(* Logix 5000 AddOnInstructionDefinition export V430_Trigger_Input_MXLSLC_102; software revision 33.01 *)

TYPE INPUT_MXLSLC_102 :
STRUCT
   Info : V430_InfoBits;
   Device_Status : V430_Device_Status;
   Fault_Code : DINT;
   Counters : V430_CodeReader_Counters;
   Read_Cycle_Report : V430_Read_Cycle_Report;
   Decode_Report : V430_Decode_Cycle_Report;
   Decode_Data : V430_MXLSLC_Str;
END_STRUCT
END_TYPE

TYPE OUTPUT_197 :
STRUCT
   Commands : V430_197_Commands;
END_STRUCT
END_TYPE

TYPE V430_197_Commands :
STRUCT
   Run_Mode : BOOL;
   Trigger : BOOL;
   Enable_Matchcode : BOOL;
   Reset_General_Fault : BOOL;
   Clear_NoRead_ReadCycle_Count : BOOL;
   Clear_MisMatch_ReadCycle_Count : BOOL;
   Clear_NoRead_Count : BOOL;
   Clear_Trigger_Count : BOOL;
   Clear_Matchcode_Count : BOOL;
   Clear_Mismatch_Count : BOOL;
   Output_1 : BOOL;
   Output_2 : BOOL;
   Output_3 : BOOL;
   Reserved1 : BOOL;
   Reserved2 : BOOL;
   Reserved3 : BOOL;
   Reserved4 : BOOL;
   Reserved5 : BOOL;
   Reserved6 : BOOL;
   Reserved7 : BOOL;
   Reserved8 : BOOL;
   Reserved9 : BOOL;
   Reserved10 : BOOL;
   Reserved11 : BOOL;
   Reserved12 : BOOL;
   Reserved13 : BOOL;
   Reserved14 : BOOL;
   Reserved15 : BOOL;
   Reserved16 : BOOL;
   Reserved17 : BOOL;
   Reserved18 : BOOL;
   Reserved19 : BOOL;
END_STRUCT
END_TYPE

TYPE V430_CodeReader_Counters :
STRUCT
   Noread_Read_Cycle_Counter : DINT;
   Mismatch_Per_Read_Cycle_Counter : DINT;
   No_Read_Counter : DINT;
   Trigger_Counter : DINT;
   Match_Code_Counter : DINT;
   Mismatch_Counter : DINT;
END_STRUCT
END_TYPE

TYPE V430_Decode_Cycle_Report :
STRUCT
   Decode_Location_Top : INT;
   Decode_Location_Left : INT;
   Decode_Location_Height : INT;
   Decode_Location_Width : INT;
   Code_Type : V430_Decode_Type;
   Pixels_Per_Element : REAL;
END_STRUCT
END_TYPE

TYPE V430_Decode_Type :
STRUCT
   Aztec : BOOL;
   MicroQR : BOOL;
   Postal_Code : BOOL;
   Code39 : BOOL;
   Codeabar : BOOL;
   I_2of5 : BOOL;
   UPC_EAN : BOOL;
   Code128_EAN128 : BOOL;
   Code93 : BOOL;
   PDF417 : BOOL;
   Pharmacode : BOOL;
   Data_Matrix : BOOL;
   QR_Code : BOOL;
   BC412 : BOOL;
   GS1_Databar : BOOL;
   GS1_Databar_Limited : BOOL;
   GS1_Databar_Expanded : BOOL;
   MicroPDF : BOOL;
   Composite : BOOL;
   Dot_Code : BOOL;
   Reserved_01 : BOOL;
   Reserved_02 : BOOL;
   Reserved_03 : BOOL;
   Reserved_04 : BOOL;
   Reserved_05 : BOOL;
   Reserved_06 : BOOL;
   Reserved_07 : BOOL;
   Reserved_08 : BOOL;
   Reserved_09 : BOOL;
   Reserved_10 : BOOL;
   Reserved_11 : BOOL;
   Reserved_12 : BOOL;
END_STRUCT
END_TYPE

TYPE V430_Device_Status :
STRUCT
   Run_Mode : BOOL;
   Trigger_Ack : BOOL;
   Exposure_Done : BOOL;
   Decoding : BOOL;
   Data_Is_Ready : BOOL;
   Read_Cycle_Pass : BOOL;
   Read_Cycle_Fail : BOOL;
   General_Fault : BOOL;
   New_Matchcode_Ack : BOOL;
   Matchcode_Enabled : BOOL;
   Image_Sensor_Calibrating : BOOL;
   Image_Sensor_Calibrated : BOOL;
   Training : BOOL;
   Train_Completed : BOOL;
   Optimizing : BOOL;
   Optimization_Complete : BOOL;
   Auto_Photometry_Enabled : BOOL;
   Auto_Photometry_Complete : BOOL;
   Output_1_Status : BOOL;
   Output_2_Status : BOOL;
   Output_3_Status : BOOL;
   Buffer_Overflow : BOOL;
   Reserved1 : BOOL;
   Reserved2 : BOOL;
   Reserved3 : BOOL;
   Reserved4 : BOOL; {access Read Only}
   Reserved5 : BOOL; {access Read Only}
   Reserved6 : BOOL; {access Read Only}
   Reserved7 : BOOL; {access Read Only}
   Reserved8 : BOOL; {access Read Only}
   Reserved9 : BOOL; {access Read Only}
   Reserved10 : BOOL; {access Read Only}
END_STRUCT
END_TYPE

TYPE V430_InfoBits :
STRUCT
   InfoBits : SINT;
   Reserved_01 : SINT;
   Reserved_02 : SINT;
   Reserved_03 : SINT;
END_STRUCT
END_TYPE

TYPE V430_MXLSLC_Str :   // string type
STRUCT
   LEN : DINT;
   DATA : SINT[184];
END_STRUCT
END_TYPE

TYPE V430_Read_Cycle_Report :
STRUCT
   Capture_Time : INT;
   Total_Decode_Time : INT;
   Total_ReadCycle_Time : INT;
   Reserved : INT;
END_STRUCT
END_TYPE

ADD_ON_INSTRUCTION V430_Trigger_Input_MXLSLC_102   (* revision 0.3, vendor OMRON *)
// Add On Instruction to trigger OMRON V430-F readers using EtherNet/IP.
// This AOI must use Input MXLSLC (102) and Output (197) assemblies
VAR_INPUT
   Execute : BOOL; {required}
   Timeout : ALIAS FOR TmrTimeout.PRE; {access None, visible}   // Maximum function execution time (milliseconds)
END_VAR
VAR_IN_OUT
   Assembly_Input : INPUT_MXLSLC_102; {required}
   Assembly_Output : OUTPUT_197; {required}
   Barcode : V430_MXLSLC_Str; {required}
   ErrorMSG : V430_MXLSLC_Str; {required}
END_VAR
VAR_OUTPUT
   Done : BOOL; {access Read Only, visible}
   Busy : BOOL; {access Read Only, visible}
   Error : BOOL; {access Read Only, visible}
   ErrorID : INT; {access Read Only, visible}
   TotalReadCycleTime : DINT; {visible}   // Function execution time (milliseconds)
   Sequencer : ALIAS FOR State; {access None}
END_VAR
VAR
   State : INT; {access None}
   Seq_at_Alarm_Timeout : INT; {access None}
   Null_Pos : INT; {access None}
   Start_Timer : BOOL; {access None}
   Alarm_Timeout : BOOL; {access None}
   FB_Running : BOOL; {access None}
   TmrTimeout : TIMER := (PRE := 30000); {access None}
   Error_Enum : V430_MXLSLC_Str[7] := ([1] := 'Read Cycle Failed.', [2] := 'Barcode Data cannot be stored in string data type. Null (0x00) character contained in Barcode Data.', [3] := 'Could not enter run mode.', [4] := 'Waiting for previous read cycle to complete. Reduce V430 Read Cycle Timeout.', [5] := 'Waiting for read cycle to start. Trigger_Acknowledge did not change state.', [6] := 'Read Cycle too long.'); {access None}
   Null_String : STRING; {access None}
   TmrOffline : TIMER := (PRE := 500); {access None}
   WaitOfflineActive : BOOL; {access None}
   WaitOfflineComplete : BOOL; {access None}
END_VAR

ROUTINE Logic   (* ladder *)
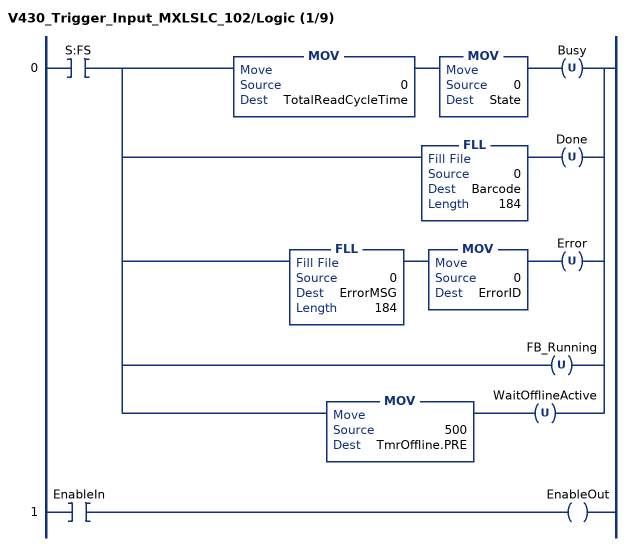
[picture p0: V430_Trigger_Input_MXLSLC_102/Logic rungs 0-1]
   0: XIC(S:FS)[MOV(0,TotalReadCycleTime) MOV(0,State) OTU(Busy) ,FLL(0,Barcode,184) OTU(Done) ,FLL(0,ErrorMSG,184) MOV(0,ErrorID) OTU(Error) ,OTU(FB_Running) ,MOV(500,TmrOffline.PRE) OTU(WaitOfflineActive) ];
   1: XIC(EnableIn)OTE(EnableOut);
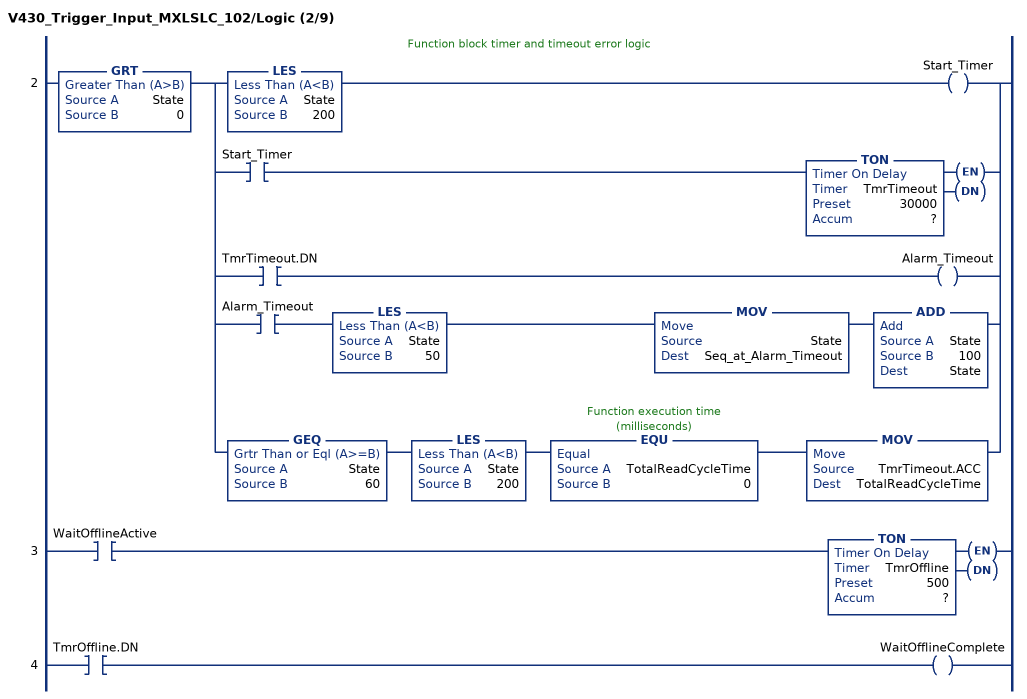
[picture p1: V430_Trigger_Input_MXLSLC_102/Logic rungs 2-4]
   // Function block timer and timeout error logic
   2: GRT(State,0)[LES(State,200) OTE(Start_Timer) ,XIC(Start_Timer) TON(TmrTimeout,?,?) ,XIC(TmrTimeout.DN) OTE(Alarm_Timeout) ,XIC(Alarm_Timeout) LES(State,50) MOV(State,Seq_at_Alarm_Timeout) ADD(State,100,State) ,GEQ(State,60) LES(State,200) EQU(TotalReadCycleTime,0) MOV(TmrTimeout.ACC,TotalReadCycleTime) ];
   3: XIC(WaitOfflineActive)TON(TmrOffline,?,?);
   4: XIC(TmrOffline.DN)OTE(WaitOfflineComplete);
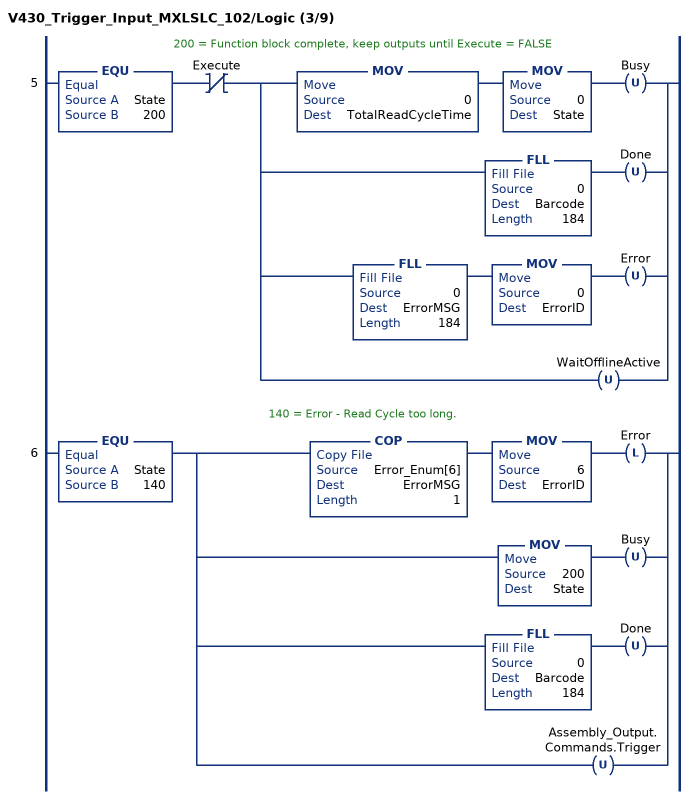
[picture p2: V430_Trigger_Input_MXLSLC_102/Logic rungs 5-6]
   // 200 = Function block complete, keep outputs until Execute = FALSE
   5: EQU(State,200)XIO(Execute)[MOV(0,TotalReadCycleTime) MOV(0,State) OTU(Busy) ,FLL(0,Barcode,184) OTU(Done) ,FLL(0,ErrorMSG,184) MOV(0,ErrorID) OTU(Error) ,OTU(WaitOfflineActive) ];
   // 140 = Error - Read Cycle too long.
   6: EQU(State,140)[COP(Error_Enum[6],ErrorMSG,1) MOV(6,ErrorID) OTL(Error) ,MOV(200,State) OTU(Busy) ,FLL(0,Barcode,184) OTU(Done) ,OTU(Assembly_Output.Commands.Trigger) ];
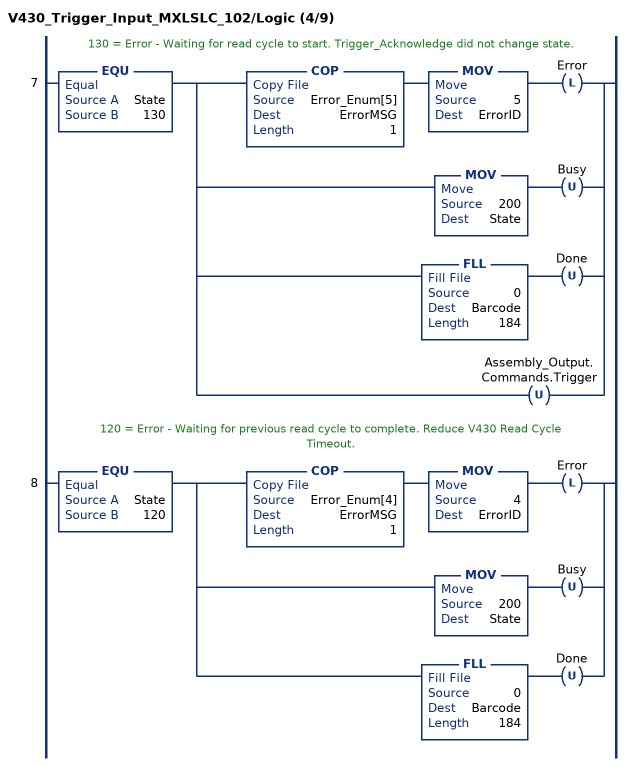
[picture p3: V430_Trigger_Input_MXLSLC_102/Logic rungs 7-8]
   // 130 = Error - Waiting for read cycle to start. Trigger_Acknowledge did not change state.
   7: EQU(State,130)[COP(Error_Enum[5],ErrorMSG,1) MOV(5,ErrorID) OTL(Error) ,MOV(200,State) OTU(Busy) ,FLL(0,Barcode,184) OTU(Done) ,OTU(Assembly_Output.Commands.Trigger) ];
   // 120 = Error - Waiting for previous read cycle to complete. Reduce V430 Read Cycle Timeout.
   8: EQU(State,120)[COP(Error_Enum[4],ErrorMSG,1) MOV(4,ErrorID) OTL(Error) ,MOV(200,State) OTU(Busy) ,FLL(0,Barcode,184) OTU(Done) ];
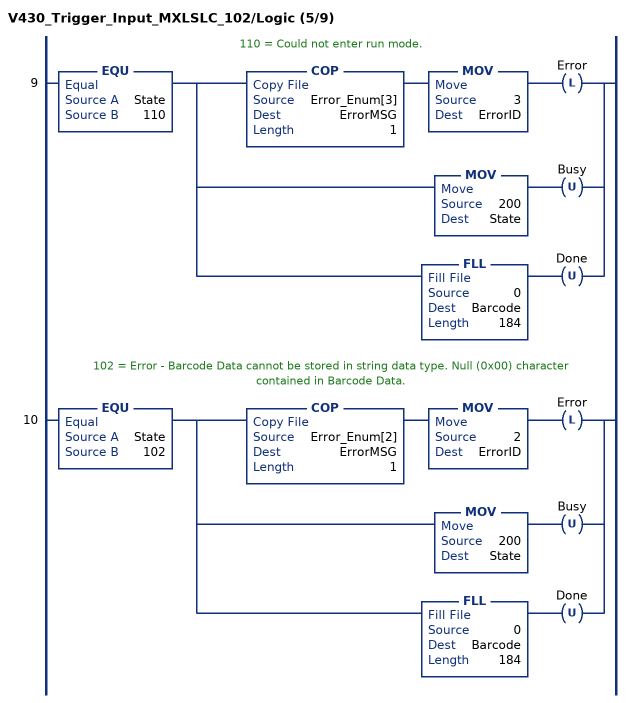
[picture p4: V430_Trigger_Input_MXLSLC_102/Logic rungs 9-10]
   // 110 = Could not enter run mode.
   9: EQU(State,110)[COP(Error_Enum[3],ErrorMSG,1) MOV(3,ErrorID) OTL(Error) ,MOV(200,State) OTU(Busy) ,FLL(0,Barcode,184) OTU(Done) ];
   // 102 = Error - Barcode Data cannot be stored in string data type. Null (0x00) character contained in Barcode Data.
   10: EQU(State,102)[COP(Error_Enum[2],ErrorMSG,1) MOV(2,ErrorID) OTL(Error) ,MOV(200,State) OTU(Busy) ,FLL(0,Barcode,184) OTU(Done) ];
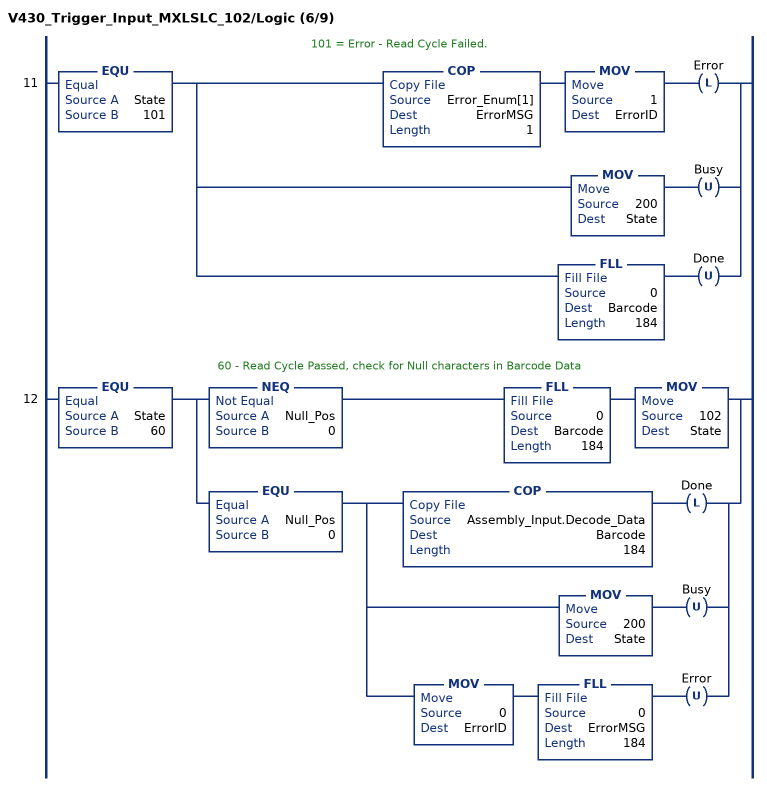
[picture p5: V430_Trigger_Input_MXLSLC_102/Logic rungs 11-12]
   // 101 = Error - Read Cycle Failed.
   11: EQU(State,101)[COP(Error_Enum[1],ErrorMSG,1) MOV(1,ErrorID) OTL(Error) ,MOV(200,State) OTU(Busy) ,FLL(0,Barcode,184) OTU(Done) ];
   // 60 - Read Cycle Passed, check for Null characters in Barcode Data
   12: EQU(State,60)[NEQ(Null_Pos,0) FLL(0,Barcode,184) MOV(102,State) ,EQU(Null_Pos,0) [COP(Assembly_Input.Decode_Data,Barcode,184) OTL(Done) ,MOV(200,State) OTU(Busy) ,MOV(0,ErrorID) FLL(0,ErrorMSG,184) OTU(Error) ] ];
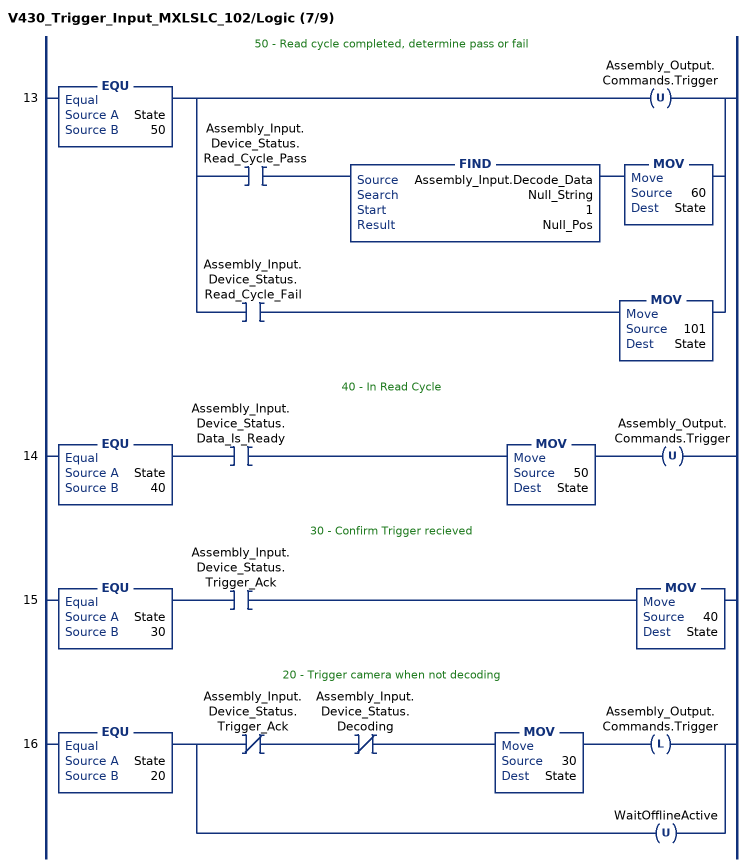
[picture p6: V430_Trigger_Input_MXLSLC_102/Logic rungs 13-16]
   // 50 - Read cycle completed, determine pass or fail
   13: EQU(State,50)[OTU(Assembly_Output.Commands.Trigger) ,XIC(Assembly_Input.Device_Status.Read_Cycle_Pass) FIND(Assembly_Input.Decode_Data,Null_String,1,Null_Pos) MOV(60,State) ,XIC(Assembly_Input.Device_Status.Read_Cycle_Fail) MOV(101,State) ];
   // 40 - In Read Cycle
   14: EQU(State,40)XIC(Assembly_Input.Device_Status.Data_Is_Ready)MOV(50,State)OTU(Assembly_Output.Commands.Trigger);
   // 30 - Confirm Trigger recieved
   15: EQU(State,30)XIC(Assembly_Input.Device_Status.Trigger_Ack)MOV(40,State);
   // 20 - Trigger camera when not decoding
   16: EQU(State,20)[XIO(Assembly_Input.Device_Status.Trigger_Ack) XIO(Assembly_Input.Device_Status.Decoding) MOV(30,State) OTL(Assembly_Output.Commands.Trigger) ,OTU(WaitOfflineActive) ];
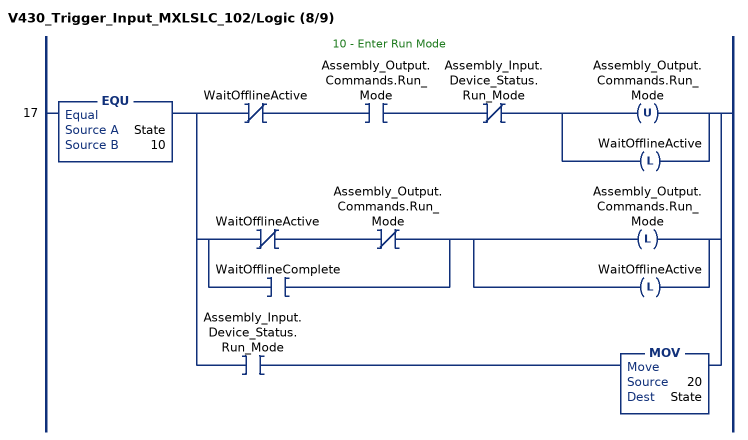
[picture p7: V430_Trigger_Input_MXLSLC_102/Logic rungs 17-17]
   // 10 - Enter Run Mode
   17: EQU(State,10)[[XIO(WaitOfflineActive) XIC(Assembly_Output.Commands.Run_Mode) XIO(Assembly_Input.Device_Status.Run_Mode) [OTU(Assembly_Output.Commands.Run_Mode) ,OTL(WaitOfflineActive) ] ,[XIO(WaitOfflineActive) XIO(Assembly_Output.Commands.Run_Mode) ,XIC(WaitOfflineComplete) ] [OTL(Assembly_Output.Commands.Run_Mode) ,OTL(WaitOfflineActive) ] ] ,XIC(Assembly_Input.Device_Status.Run_Mode) MOV(20,State) ];
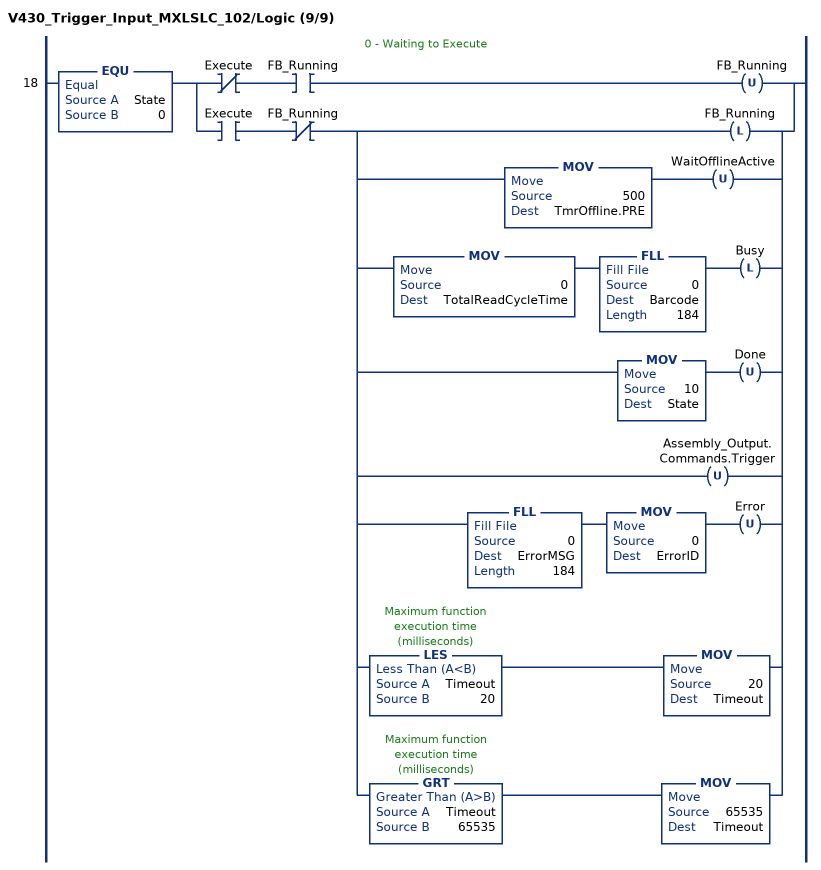
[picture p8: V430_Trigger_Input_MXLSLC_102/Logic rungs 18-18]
   // 0 - Waiting to Execute
   18: EQU(State,0)[XIO(Execute) XIC(FB_Running) OTU(FB_Running) ,XIC(Execute) XIO(FB_Running) [OTL(FB_Running) ,MOV(500,TmrOffline.PRE) OTU(WaitOfflineActive) ,MOV(0,TotalReadCycleTime) FLL(0,Barcode,184) OTL(Busy) ,MOV(10,State) OTU(Done) ,OTU(Assembly_Output.Commands.Trigger) ,FLL(0,ErrorMSG,184) MOV(0,ErrorID) OTU(Error) ,LES(Timeout,20) MOV(20,Timeout) ,GRT(Timeout,65535) MOV(65535,Timeout) ] ];
END_ROUTINE
END_ADD_ON_INSTRUCTION
